TYPE ST_AXIS_DATA :
STRUCT
	AXIS_REF		:	AXIS_REF;
	
	//======== input =================
	bHome			:	BOOL;
	bHomeCam		:	BOOL;
	bEnable			:	BOOL;
	bStop			:	BOOL;
	// jog
	bJogForward		: 	BOOL;
    bJogBackward	: 	BOOL;
    eMode			: 	E_JogMode := E_JogMode.MC_JOGMODE_CONTINOUS;
	// reset
	bResetAxis		:	BOOL;
	// setPos
	bSetPos			:	BOOL;
	// Move
	bMoveAbs		:	BOOL;
	bMoveVelo		:	BOOL;
	rPosition		:	REAL;
	rVelocity		:	REAL;
	rAcc			:	LREAL;
	rDec			:	LREAL;
	rJerk			:	LREAL;
	// GearIn
	bGearIn			:	BOOL;
	bGearOut		:	BOOL;
	refMaster		:	REFERENCE TO AXIS_REF;
	RatioNumerator	:	LREAL := 1.0;
	RatioDenominator:	UINT := 1;
	//========= status ================
	bEnabled		:	BOOL;// 已经使能
END_STRUCT
END_TYPE
